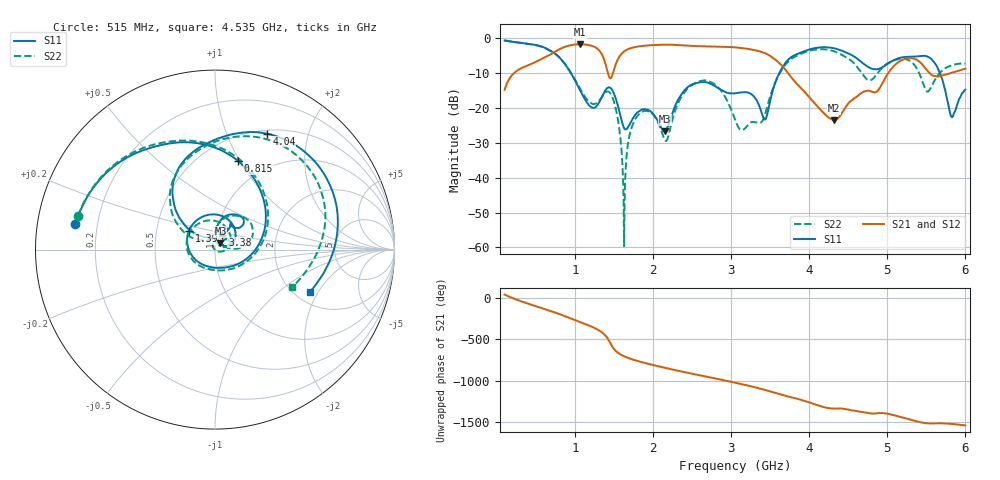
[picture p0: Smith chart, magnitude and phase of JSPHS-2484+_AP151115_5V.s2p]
!Mini-Circuits Laboratory
!S-Parameters
!Run/Lot/Date Code:MF33450/NA/1551
!Fixture/SN/Due: 90-4-20-21/70546/03/17/16
!Connection:PORT<IN> - pin<1>; PORT<OUT> - pin<7>;PORT<BIAS> - pin<4>;
!Tested With:PORT EXTENTION
!Network Analyzer:AG E5071C/74883/05/12/16
!Created: 01-07-2016 at 14:09:44
!MODEL: JSPHS-2484+
!S/N: V=5V
# MHZ S DB R 50
!Frequency  S11 dB  S11 DEG  S21 dB  S21 DEG  S12 dB  S12 DEG  S22 dB  S22 DEG
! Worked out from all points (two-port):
!   1181 points, 100 MHz to 6 GHz, reference 50 ohm
!   highest |S21| = -1.76 dB at 1.06 GHz (marker M1); lowest = -23.5 dB at 4.315 GHz (marker M2)
!   |S21| within 3 dB of the highest: 679.3 MHz to 1.347 GHz (667.9 MHz wide, 65.9 % of centre); 1.587 GHz to 3.475 GHz (1.889 GHz wide, 74.6 % of centre)
!   lowest |S11| = -26.7 dB at 2.15 GHz (marker M3), VSWR 1.10, Z = 53 + j3.67 ohm
!   |S11| at or under -10 dB: 948.4 MHz to 3.618 GHz (2.669 GHz wide, 117 % of centre); 5.673 GHz to end of sweep
!   |S22| runs from -59.6 to -0.7 dB; largest |S21 - S12| = 0.001
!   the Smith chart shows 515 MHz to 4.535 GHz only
!   S11 on the Smith chart (normalised r, x): 515 MHz: 0.12, +0.09; 815 MHz: 0.74, +0.98; 1.39 GHz: 0.73, +0.16; 3.38 GHz: 1.07, +0.18; 4.04 GHz: 0.54, +1.40; 4.535 GHz: 2.40, -1.70
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100  -0.66 -48.1  -14.81 41.6  -14.80 41.6  -0.66 -48.1
515  -2.04 169.7  -6.62 -102.7  -6.62 -102.7  -2.09 166.3
815  -5.84 75.4  -3.02 160.4  -3.02 160.4  -5.85 72.0
1060  -14.65 -15.3  -1.76 72.1  -1.76 72.1  -14.23 -17.9
1085  -15.74 -25.3  -1.77 63.1  -1.77 63.1  -15.22 -27.9
1250  -19.95 -107.0  -2.49 -1.7  -2.49 -1.7  -18.89 -104.0
1390  -14.94 144.2  -7.25 -93.5  -7.25 -93.5  -15.57 158.1
1630  -25.80 22.1  -3.80 15.2  -3.80 15.2  -59.64 -134.6
1770  -22.05 45.3  -2.55 -32.9  -2.55 -32.9  -23.27 77.6
2070  -24.02 18.2  -1.91 -106.1  -1.91 -106.1  -24.39 13.7
2150  -26.74 48.6  -1.86 -123.7  -1.86 -123.8  -29.15 37.5
2600  -12.67 55.0  -2.30 145.1  -2.30 145.1  -12.34 48.1
3050  -15.83 56.0  -2.64 56.1  -2.64 56.1  -23.33 10.5
3380  -20.64 63.4  -3.87 -17.6  -3.87 -17.7  -24.17 115.5
4035  -3.03 66.9  -17.81 166.0  -17.80 165.9  -3.45 68.1
4040  -3.00 66.1  -17.94 164.4  -17.94 164.3  -3.43 67.3
4315  -2.88 19.1  -23.50 102.7  -23.49 102.7  -3.75 19.0
4535  -4.74 -23.9  -18.00 83.3  -17.99 83.6  -6.41 -25.7
5020  -7.14 147.0  -9.73 36.9  -9.74 36.8  -6.98 112.6
5500  -5.16 21.8  -8.97 -74.9  -8.97 -74.9  -15.09 52.5
5820  -22.45 -1.9  -9.95 -82.8  -9.95 -82.7  -7.83 74.4
6000  -14.75 40.5  -8.74 -101.6  -8.74 -101.6  -7.28 60.6
